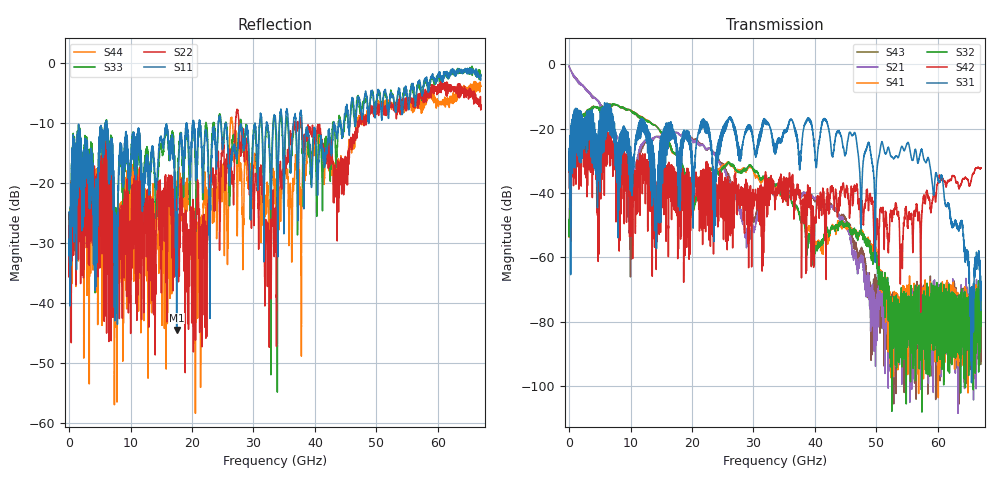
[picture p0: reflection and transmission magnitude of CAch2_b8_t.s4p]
!Agilent Technologies,N5247A,US51170199,A.09.90.13
!Agilent N5247A: A.09.90.13
!Date: Tuesday, October 23, 2018 13:12:43
!Correction: S11(Full 4 Port(1,2,3,4))
!S12(Full 4 Port(1,2,3,4))
!S13(Full 4 Port(1,2,3,4))
!S14(Full 4 Port(1,2,3,4))
!S21(Full 4 Port(1,2,3,4))
!S22(Full 4 Port(1,2,3,4))
!S23(Full 4 Port(1,2,3,4))
!S24(Full 4 Port(1,2,3,4))
!S31(Full 4 Port(1,2,3,4))
!S32(Full 4 Port(1,2,3,4))
!S33(Full 4 Port(1,2,3,4))
!S34(Full 4 Port(1,2,3,4))
!S41(Full 4 Port(1,2,3,4))
!S42(Full 4 Port(1,2,3,4))
!S43(Full 4 Port(1,2,3,4))
!S44(Full 4 Port(1,2,3,4))
!S4P File: Measurements: <S11,S12,S13,S14>,
!<S21,S22,S23,S24>,
!<S31,S32,S33,S34>,
!<S41,S42,S43,S44>:
# Hz S  dB  R 50
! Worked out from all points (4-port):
!   6701 points, 10 MHz to 67 GHz, reference 50 ohm
!   strongest paths, dB at 10 MHz, 16.76 GHz, 33.51 GHz, 50.25 GHz, 67 GHz:
!     S31: -33.0, -22.8, -25.8, -30.2, -76.4
!     S42: -33.5, -33.4, -44.1, -52.6, -32.1
!     S32: -48.4, -26.6, -38.0, -63.2, -78.1
!     S41: -48.2, -26.8, -38.0, -60.9, -75.7
!     S21: -0.6, -21.4, -40.7, -72.0, -74.1
!     S43: -0.5, -21.5, -40.2, -68.9, -92.2
!   lowest |S11| = -44.5 dB at 17.51 GHz (marker M1), VSWR 1.01, Z = 50.6 + j0.129 ohm
!   |S11| at or under -10 dB: start of sweep to 5.972 GHz; 6.104 GHz to 20.15 GHz (14.05 GHz wide, 107 % of centre); 24.68 GHz to 31.02 GHz (6.332 GHz wide, 22.7 % of centre)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
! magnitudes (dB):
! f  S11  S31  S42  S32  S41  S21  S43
! 10 MHz  -24.9  -33.0  -33.5  -48.4  -48.2  -0.6  -0.5
! 1.89 GHz  -18.0  -30.6  -34.1  -16.8  -16.8  -5.9  -5.9
! 9.939 GHz  -18.7  -34.7  -34.1  -14.2  -14.2  -35.6  -53.8
! 12.01 GHz  -21.6  -18.9  -32.7  -16.8  -16.6  -24.3  -24.8
! 17.51 GHz  -44.5  -25.0  -33.8  -28.4  -28.5  -21.1  -21.2
! 55.1 GHz  -6.0  -24.3  -50.6  -78.2  -73.1  -76.6  -72.4
! 67 GHz  -2.0  -76.4  -32.1  -78.1  -75.7  -74.1  -92.2
